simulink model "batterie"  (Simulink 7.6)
settings: Solver=ode23tb  StartTime=0.0  StopTime=N  MaxStep=0.1  RelTol=1e-4
InitFcn:
  | N=2500; % durée de la simulation
  | 
  | switch_on=80;
  | switch_off=40;
  | 
  | positive_SlewRate=80;
  | negative_SlewRate=-80;
  | 
  | negative_torque=-200;
StopFcn:
  | close all, clc
  | 
  | load batt.mat
  | plotyy(x(1,:),x(2,:), x(1,:),x(3,:))
  | grid
  | title('Tension batterie et état de charge')
  | xlabel('temps')
  | axis([0 N 100 300])
  | delete *.mat, clear all
undefined symbols (not defined in the file or in its folder): Hydride, Metal, Nickel
libraries: powerlib x2, electricdrivelib x1, simulink x1

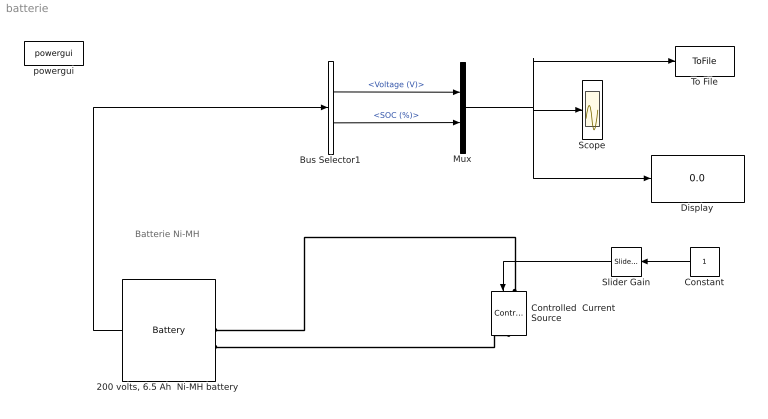
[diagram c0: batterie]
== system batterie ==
  note: Batterie Ni-MH
  "200 volts, 6.5 Ah  Ni-MH battery " : electricdrivelib/Extra Sources/Battery  DialogController=POWERSYS.PowerSysDialog  SystemSampleTime=-1  BatType=Nickel-Metal-Hydride  ShowDetailedParameters=off  NomV=200  NomQ=6.5  SOC=100  PresetModel=on  MaxQ=7  FullV=235.5932  Dis_rate=1.3  R=0.30769  Normal_OP=6.25  expZone="[216.9492           1.3]"  Dis_Char=off  current=50  Units=Ampere-hour  Batt_Tr=30
  Bus Selector1 : BusSelector  OutputSignals=Voltage (V),SOC (%)
  Constant : Constant
  Controlled  Current Source : powerlib/Electrical Sources/Controlled Current Source  DialogController=POWERSYS.PowerSysDialog  SystemSampleTime=-1  Initialize=on  Source_Type=AC  Amplitude=0  Phase=0  Frequency=0  Measurements=None
  Display : Display
  Mux : Mux  Inputs=2
  Scope : Scope
  Slider Gain : simulink/Math Operations/Slider Gain  SystemSampleTime=-1  low=0  gain=10  high=20
  To File : ToFile  Filename=batt.mat  MatrixName=x
  powergui : powerlib/powergui  SystemSampleTime=-1  SimulationMode=Continuous  SampleTime=0.001  frequency=60  SPID=off  DisableSnubberDevices=off  DisableRonSwitches=off  DisableVfSwitches=off  SwTol=0  Interpol=off  frequencyindice=0  echomessages=off  HookPort=off  DisplayEquations=off  FunctionMessages=off  EnableUseOfTLC=off  x0status=blocks  RestoreLinks=warning  ResistiveCurrentMeasurement=off  Frange=[0:2:500]  Ylog=off  Xlog=on  ShowGrid=off  save=off  variable=ZData  ZoomFFT=on  StartTime=0.0  cycles=1  DisplayStyle=1  fundamental=60  FreqAxis=off  MaxFrequency=1000  frequencyindicesteady=1  RmsSteady=1  display=off  Ts=0  methode=off
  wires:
  "200 volts, 6.5 Ah  Ni-MH battery "/1 -> Bus Selector1/1
  Bus Selector1/1 -> Mux/1  "<Voltage (V)>"
  Bus Selector1/2 -> Mux/2  "<SOC (%)>"
  Mux/1 -> Scope/1, Display/1, To File/1
  Constant/1 -> Slider Gain/1
  Slider Gain/1 -> Controlled  Current Source/1
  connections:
  "200 volts, 6.5 Ah  Ni-MH battery "/LConn2 -- Controlled  Current Source/RConn1
  Controlled  Current Source/LConn1 -- "200 volts, 6.5 Ah  Ni-MH battery "/LConn1
